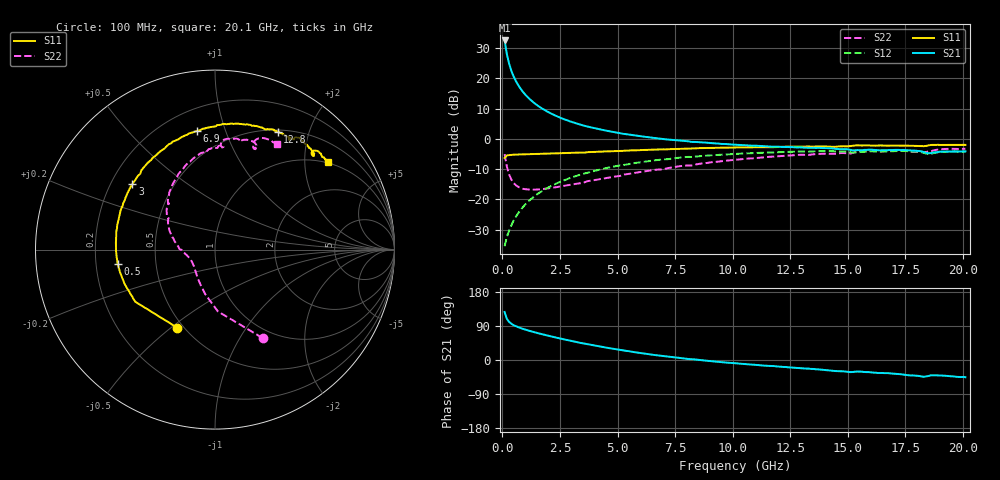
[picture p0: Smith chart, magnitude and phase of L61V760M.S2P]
!  Infineon Technologies AG
! BFR380L3 , PF131585-7, No.6, Th 09.10.01, soldered on pcb-board, measured with PP GSG850
!  Vce=1.75 V,  Ic=60.0 mA
! Common Emitter S-Parameters:  15. November 2001
#  GHz  S  MA  R  50
! f  S11  S21  S12  S22
! GHz  Mag  Ang  Mag  Ang  Mag  Ang  Mag  Ang
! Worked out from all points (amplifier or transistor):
!   201 points, 100 MHz to 20.1 GHz, reference 50 ohm
!   highest |S21| = 32.5 dB at 100 MHz (marker M1)
!   |S21| within 3 dB of that: start of sweep to 165.1 MHz
!   unconditionally stable (mu >= 1): 695 MHz to 4.357 GHz; 18.25 GHz to 18.61 GHz
!   at 3.4 GHz: K = 1.02, MAG = 7.4 dB, |S12| = -11.8 dB
!   at 10.1 GHz: K = 0.97, MSG = 1.5 dB, |S12| = -5.0 dB
!   at 20.1 GHz: K = 0.99, MSG = 0.0 dB, |S12| = -4.2 dB
!   S11 on the Smith chart (normalised r, x): 100 MHz: 0.46, -0.52; 500 MHz: 0.29, -0.07; 3 GHz: 0.29, +0.32; 6.9 GHz: 0.33, +0.80; 12.8 GHz: 0.53, +1.54; 20.1 GHz: 0.98, +2.59
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0.1  0.4831 -115.9  41.96 126.5  0.01694 57.4  0.5591 -61.7
0.2  0.5309 -146.8  24.69 108.3  0.02426 58.2  0.3446 -87.3
0.3  0.5388 -159.0  17.11 100.3  0.03107 62.1  0.2551 -102.1
0.4  0.5442 -166.7  13.04 95.4  0.0379 64.9  0.2102 -112.8
0.5  0.548 -171.7  10.51 91.7  0.04527 67.2  0.1855 -121.1
0.6  0.5495 -175.8  8.8 88.9  0.05256 68.5  0.1703 -127.7
0.7  0.5512 -178.9  7.577 86.3  0.05997 69.5  0.1607 -133.3
0.8  0.5521 178.4  6.645 84.1  0.0676 70.1  0.1543 -137.9
1  0.5543 173.6  5.348 80.1  0.08267 70.4  0.1475 -145.0
1.2  0.5593 169.6  4.48 76.6  0.09791 70.2  0.1455 -150.4
1.5  0.562 164.2  3.614 71.6  0.1205 69.2  0.1457 -156.5
1.9  0.5694 157.7  2.891 65.4  0.1506 67.1  0.1508 -162.7
3  0.5868 141.6  1.907 50.2  0.2295 59.8  0.1756 -175.5
3.5  0.5934 135.0  1.668 44.0  0.2643 56.1  0.1874 -179.9
5.1  0.6295 116.5  1.24 26.5  0.3647 43.9  0.2442 164.0
6.8  0.6671 99.7  1.011 11.8  0.4505 31.6  0.312 146.6
6.9  0.6686 98.8  0.9984 11.0  0.4542 30.8  0.3122 145.7
10.1  0.7202 75.8  0.799 -8.5  0.5627 9.7  0.4502 119.3
12.8  0.7426 61.9  0.7202 -21.2  0.6157 -6.8  0.5429 98.5
13.5  0.7461 58.8  0.7123 -23.6  0.6202 -10.6  0.5532 94.3
16.8  0.773 47.0  0.6536 -35.0  0.6231 -26.1  0.634 74.8
20.1  0.7949 37.9  0.62 -45.4  0.6156 -39.4  0.685 59.5
